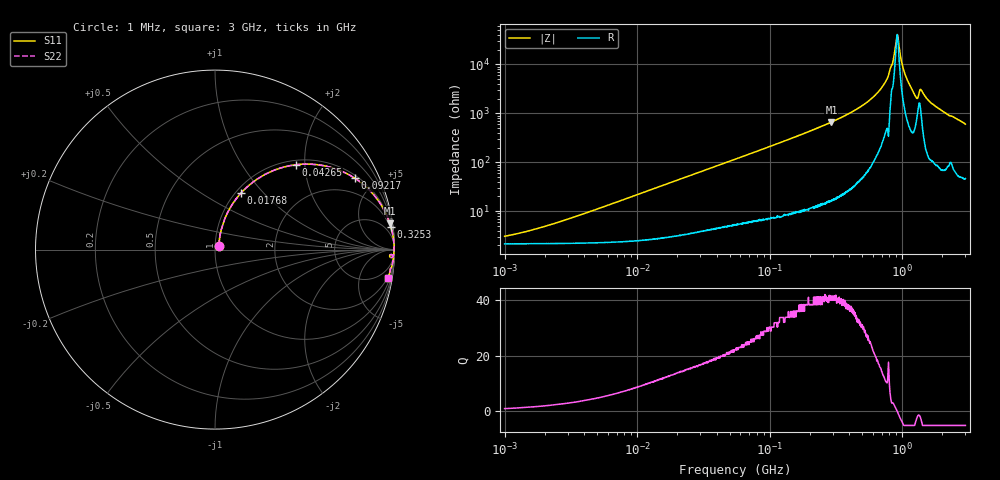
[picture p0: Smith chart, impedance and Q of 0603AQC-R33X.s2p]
!s-Parameter Generated by FASTRON Sdn. Bhd.
!FASTRON P/N : 0603AQC-R33X
!Keysight Technologies: E4991B_MY54100416_A.01.15
!Date: Thu Jun 25 14:07:51 2026
!Version  :Rev00  Thu Jun 25 14:07:51 2026
!Data & Calibration Information:
!Freq  S11  S21  S12  S22
!PortZ  Port1:50+j0  Port2:50+j0
!When reading reference impedance value at option line is always used.
! Remarks : This data is being provided solely for informational purposes.
# Hz S dB R 50
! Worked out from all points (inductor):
!   1601 points, 1 MHz to 3 GHz, reference 50 ohm
!   read as one part in series: L = 345 nH near 3.022 MHz
!   highest Q = 41.2 at 292.8 MHz (marker M1), where L = 362 nH
!   self-resonance near 916.4 MHz
!   S11 on the Smith chart (normalised r, x): 1 MHz: 1.04, +0.04; 17.68 MHz: 1.06, +0.76; 42.65 MHz: 1.09, +1.80; 92.17 MHz: 1.13, +3.85; 325.3 MHz: 1, +15; 3 GHz: 2, -12
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1000000  -30.50 44.3  -0.19 -1.2  -0.19 -1.2  -30.50 44.3
3804036  -21.60 70.4  -0.22 -4.6  -0.22 -4.6  -21.60 70.4
1.447069e7  -10.70 68.1  -0.62 -16.8  -0.62 -16.8  -10.70 68.1
1.767735e7  -9.21 65.3  -0.81 -20.2  -0.81 -20.2  -9.21 65.3
4.264819e7  -3.70 46.4  -2.79 -40.7  -2.79 -40.7  -3.70 46.4
5.504702e7  -2.61 39.7  -3.88 -47.7  -3.88 -47.7  -2.61 39.7
9.216659e7  -1.15 27.0  -6.87 -61.0  -6.87 -61.0  -1.15 27.0
2.083556e8  -0.26 12.4  -13.30 -76.1  -13.30 -76.1  -0.26 12.4
2.92808e8  -0.13 8.5  -16.60 -80.1  -16.60 -80.1  -0.13 8.5
3.252521e8  -0.10 7.5  -17.70 -81.1  -17.70 -81.1  -0.10 7.5
5.899715e8  -0.03 2.8  -26.20 -84.7  -26.20 -84.7  -0.03 2.8
7.135306e8  -0.02 1.6  -31.20 -84.1  -31.20 -84.1  -0.02 1.6
7.925923e8  -0.01 0.9  -36.10 -85.3  -36.10 -85.3  -0.01 0.9
8.501091e8  -0.02 0.5  -41.00 -71.4  -41.00 -71.4  -0.02 0.5
8.982141e8  -0.02 0.1  -49.10 -44.4  -49.10 -44.4  -0.02 0.1
9.209708e8  -0.02 -0.0  -52.20 6.0  -52.20 6.0  -0.02 -0.0
9.443041e8  -0.02 -0.2  -48.10 52.1  -48.10 52.1  -0.02 -0.2
1.0437e9  -0.02 -0.8  -36.50 78.8  -36.50 78.8  -0.02 -0.8
1.255985e9  -0.10 -2.4  -27.20 74.0  -27.20 74.0  -0.10 -2.4
1.402151e9  -0.08 -1.9  -29.40 73.2  -29.40 73.2  -0.08 -1.9
1.791767e9  -0.06 -4.1  -22.90 82.3  -22.90 82.3  -0.06 -4.1
3e9  -0.22 -9.3  -15.80 76.3  -15.80 76.3  -0.22 -9.3
